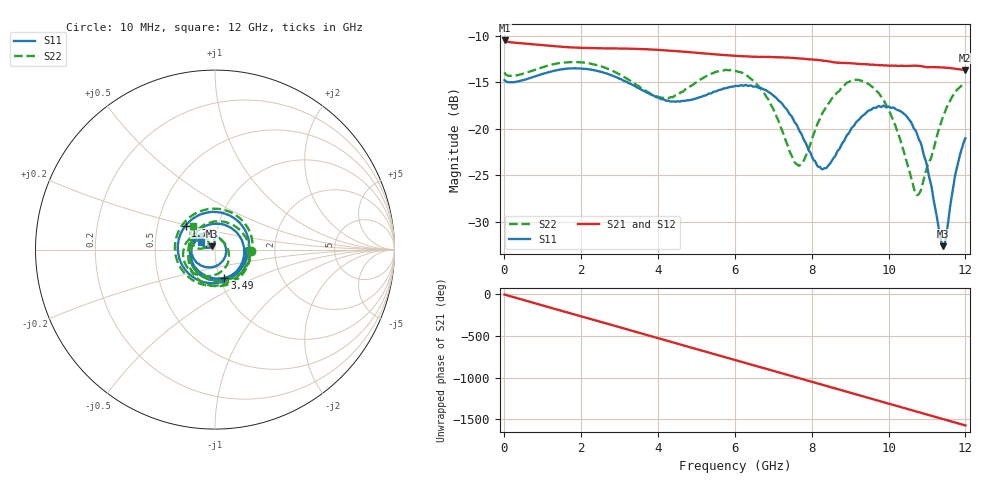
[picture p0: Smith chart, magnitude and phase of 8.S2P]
!Agilent Technologies,E5071C,MY46316741,A.11.02
!Date: Fri Apr 15 15:50:03 2022
!Data & Calibration Information:
!Freq	S11:SOLT2(ON)	S21:SOLT2(ON)	S12:SOLT2(ON)	S22:SOLT2(ON)
!PortZ  Port1:50+j0  Port2:50+j0
!Above PortZ is port z conversion or system Z0 setting when saving the data.
!When reading, reference impedance value at option line is always used.
# Hz S dB R 50
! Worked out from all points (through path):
!   1200 points, 10 MHz to 12 GHz, reference 50 ohm
!   highest |S21| = -10.47 dB at 10 MHz (marker M1); lowest = -13.6 dB at 11.99 GHz (marker M2)
!   group delay of S21, straight-line fit = 363 ps
!   lowest |S11| = -32.6 dB at 11.42 GHz (marker M3), VSWR 1.05, Z = 48.5 + j1.74 ohm
!   |S11| at or under -10 dB: start of sweep to end of sweep
!   |S22| runs from -27.1 to -12.8 dB; largest |S21 - S12| = 0.0018
!   S11 on the Smith chart (normalised r, x): 10 MHz: 1.45, -0.02; 1.71 GHz: 0.70, +0.19; 3.49 GHz: 1.05, -0.34; 12 GHz: 0.85, +0.07
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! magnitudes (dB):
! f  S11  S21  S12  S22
! 10 MHz  -14.8  -10.5  -10.5  -13.9
! 1.71 GHz  -13.5  -11.2  -11.2  -12.8
! 2.01 GHz  -13.5  -11.3  -11.3  -12.8
! 3.49 GHz  -15.6  -11.4  -11.4  -15.4
! 4.01 GHz  -16.6  -11.5  -11.5  -16.6
! 6.01 GHz  -15.4  -12.1  -12.1  -13.8
! 6.81 GHz  -15.8  -12.2  -12.2  -16.5
! 7.6 GHz  -19.5  -12.4  -12.4  -23.8
! 7.77 GHz  -20.9  -12.4  -12.4  -23.6
! 8.01 GHz  -23.0  -12.5  -12.5  -21.1
! 8.38 GHz  -24.2  -12.7  -12.7  -17.6
! 9.04 GHz  -19.9  -12.9  -12.9  -14.8
! 9.59 GHz  -17.8  -13.1  -13.1  -15.5
! 10.01 GHz  -17.6  -13.2  -13.2  -18.0
! 10.42 GHz  -18.4  -13.2  -13.2  -22.8
! 10.75 GHz  -20.7  -13.2  -13.2  -27.1
! 11 GHz  -24.0  -13.4  -13.4  -24.1
! 11.42 GHz  -32.6  -13.4  -13.4  -18.6
! 11.5 GHz  -31.6  -13.4  -13.4  -17.8
! 11.76 GHz  -24.5  -13.5  -13.5  -15.9
! 11.99 GHz  -21.1  -13.6  -13.6  -15.1
! 12 GHz  -21.0  -13.6  -13.6  -15.1
